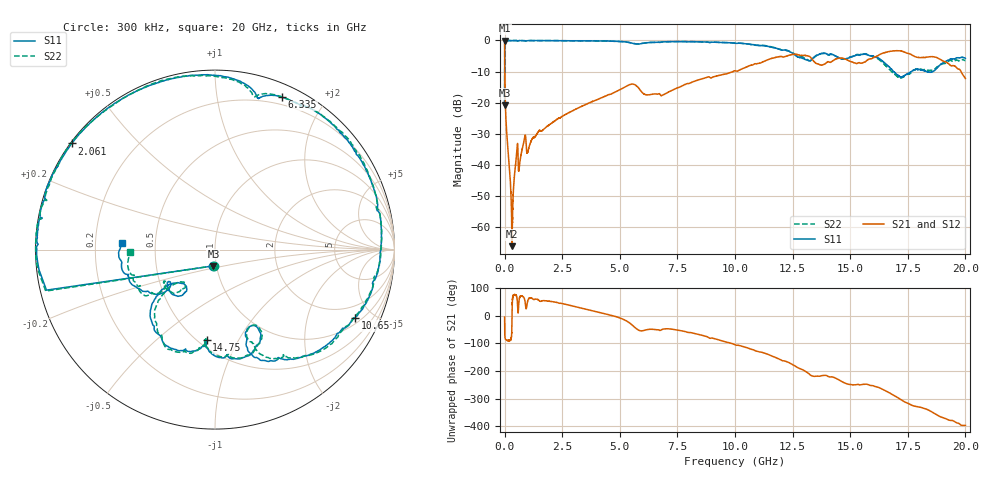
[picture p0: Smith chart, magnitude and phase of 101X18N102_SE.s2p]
!{101X18N102_SE}
!Johanson Technology Inc.
!www.johansontechnology.com
!Test Board Conditions:
!Substrate Type  RO4350B
!Substrate Thickness  21 mil
!Substrate Dk  3.66
!TL Type: GCPW
!TL Trace Width  40 mil
!TL Gap  20 mil
!PART MODE SINGLE ENDED (AKA BYPASS)
!DUT TOPOLOGY	SERIES-SHUNT
!Mounting Pad LxW  120x40 mil
! Created Wed Oct 27 11:11:44 2021
# hz S ma R 50
! 2 Port Network Data from SP1.SP block
! freq  magS11  angS11  magS21  angS21  magS12  angS12  magS22  angS22
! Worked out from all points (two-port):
!   20001 points, 300 kHz to 20 GHz, reference 50 ohm
!   highest |S21| = -0.06 dB at 300 kHz (marker M1); lowest = -66.1 dB at 321.3 MHz (marker M2)
!   |S21| within 3 dB of the highest: start of sweep to 3.318 MHz
!   lowest |S11| = -20.8 dB at 300 kHz (marker M3), VSWR 1.20, Z = 48.3 - j8.85 ohm
!   |S11| at or under -10 dB: 16.88 GHz to 17.66 GHz (773.7 MHz wide, 4.48 % of centre); 18.31 GHz to 18.59 GHz (273.6 MHz wide, 1.48 % of centre); 18.58963 GHz to 18.5922 GHz (2.572 MHz wide, 0.0138 % of centre)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
!   |S22| runs from -20.9 to 0.0 dB; largest |S21 - S12| = 0.018
!   S11 on the Smith chart (normalised r, x): 300 kHz: 0.97, -0.18; 2.061 GHz: 0.00, +0.33; 6.335 GHz: 0.12, +1.52; 10.65 GHz: 1.29, -3.93; 14.75 GHz: 0.55, -0.75; 20 GHz: 0.32, +0.03
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300000  0.09121 -95.6  0.9936 -5.1  0.9957 -5.3  0.09026 -94.3
1.023e8  0.9927 179.9  0.02884 -89.3  0.0289 -89.3  0.9996 179.9
2.473e8  0.9918 176.1  0.005628 -88.6  0.005553 -88.5  1 176.2
3.213e8  0.9937 174.5  0.0004948 -18.7  0.0006788 -15.3  0.9999 174.6
4.923e8  0.9944 170.9  0.0116 74.2  0.01153 73.5  0.9995 171.2
8.333e8  0.9947 164.8  0.02343 65.6  0.02358 65.8  0.9906 164.8
2.0613e9  0.9931 143.4  0.04753 50.7  0.04751 50.8  0.9964 143.4
3.3343e9  0.9852 119.8  0.08697 27.3  0.08716 27.3  0.9854 118.4
5.4893e9  0.911 76.5  0.1982 -30.6  0.1985 -30.5  0.915 78.1
6.3353e9  0.9278 66.3  0.1352 -49.1  0.1351 -49.4  0.9275 67.2
6.6673e9  0.9353 60.2  0.1379 -50.8  0.1381 -51.2  0.9358 61.2
8.4773e9  0.9486 23.0  0.2365 -69.1  0.235 -68.9  0.9515 24.0
1.00003e10  0.9015 -11.0  0.3239 -105.3  0.3265 -105.2  0.9031 -9.1
1.06493e10  0.8667 -26.0  0.3958 -119.8  0.3941 -120.3  0.8685 -24.6
1.25313e10  0.6101 -71.2  0.5984 -178.2  0.5945 -177.3  0.6221 -67.1
1.33343e10  0.5021 -61.3  0.5024 142.4  0.5046 142.7  0.4932 -60.7
1.47523e10  0.5058 -95.3  0.5081 116.8  0.5095 116.8  0.5027 -95.7
1.55943e10  0.6004 -113.2  0.4454 111.8  0.4437 110.9  0.6112 -112.7
1.66673e10  0.3828 -142.4  0.6607 82.4  0.6633 83.7  0.3534 -140.6
1.73673e10  0.2754 -124.8  0.6485 48.2  0.6504 48.5  0.2679 -128.2
1.85843e10  0.3157 -141.3  0.5492 10.5  0.5495 10.3  0.3371 -144.4
2e10  0.5153 175.7  0.2449 -36.5  0.2445 -37.1  0.4748 -178.8
